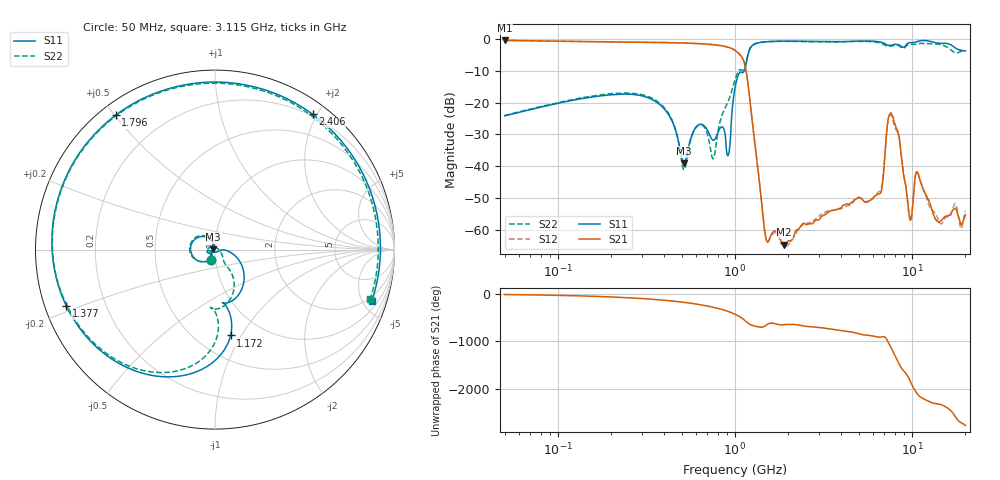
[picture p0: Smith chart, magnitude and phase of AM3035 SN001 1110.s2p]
# Hz S DB R 50
!freq MagS11 AngS11 MagS21 AngS21 MagS12 AngS12 MagS22 AngS22
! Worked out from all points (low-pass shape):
!   1601 points, 50 MHz to 20.05 GHz, reference 50 ohm
!   highest |S21| = -0.38 dB at 50 MHz (marker M1); lowest = -64.7 dB at 1.9 GHz (marker M2)
!   |S21| within 3 dB of the highest: start of sweep to 995.3 MHz
!   lowest |S11| = -39.2 dB at 515.9 MHz (marker M3), VSWR 1.02, Z = 48.9 + j0.261 ohm
!   |S11| at or under -10 dB: start of sweep to 1.129 GHz
!   |S22| runs from -41.2 to -0.6 dB; largest |S21 - S12| = 0.014
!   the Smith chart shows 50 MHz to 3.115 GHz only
!   S11 on the Smith chart (normalised r, x): 50 MHz: 0.95, -0.11; 1.172 GHz: 0.72, -0.90; 1.377 GHz: 0.06, -0.18; 1.796 GHz: 0.04, +0.50; 2.406 GHz: 0.17, +1.94; 3.115 GHz: 1.57, -5.83
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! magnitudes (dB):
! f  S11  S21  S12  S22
! 50 MHz  -24.2  -0.4  -0.4  -24.1
! 135.9 MHz  -18.7  -0.7  -0.7  -18.5
! 369.6 MHz  -20.3  -1.0  -1.0  -19.9
! 515.9 MHz  -39.2  -1.2  -1.2  -41.2
! 631.6 MHz  -26.8  -1.4  -1.4  -27.0
! 756 MHz  -31.9  -1.7  -1.7  -37.6
! 918.6 MHz  -36.4  -2.5  -2.5  -19.4
! 1.005 GHz  -14.9  -3.6  -3.6  -12.5
! 1.172 GHz  -6.3  -11.9  -11.9  -5.9
! 1.377 GHz  -1.1  -45.2  -45.1  -1.0
! 1.512 GHz  -0.8  -63.6  -63.5  -0.8
! 1.796 GHz  -0.6  -62.8  -63.7  -0.7
! 1.9 GHz  -0.6  -64.7  -65.1  -0.7
! 2.406 GHz  -0.6  -58.3  -58.6  -0.7
! 2.722 GHz  -0.7  -58.2  -57.6  -0.8
! 3.115 GHz  -0.7  -55.7  -54.8  -0.8
! 6.566 GHz  -0.8  -48.7  -48.0  -1.1
! 7.402 GHz  -1.9  -24.3  -24.7  -2.3
! 9.766 GHz  -1.1  -56.8  -57.1  -1.6
! 10.73 GHz  -0.7  -41.8  -41.9  -1.5
! 14.47 GHz  -1.3  -57.4  -58.1  -1.7
! 20.05 GHz  -3.7  -55.4  -54.1  -3.6
